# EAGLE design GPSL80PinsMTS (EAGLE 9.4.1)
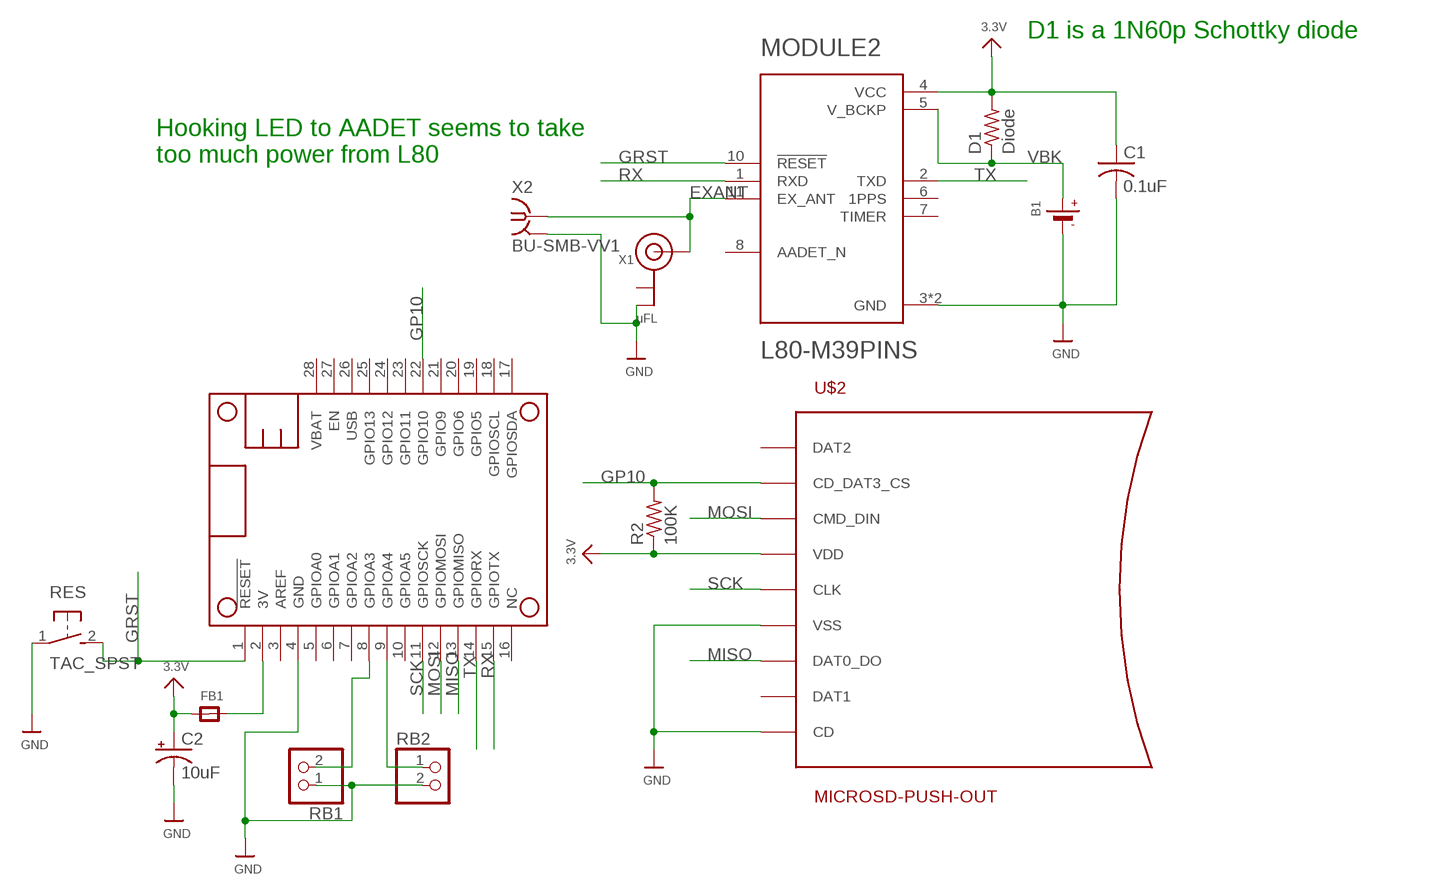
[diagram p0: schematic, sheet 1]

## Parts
B1  MICROBUILDER_BATTERYCR1220_2  [MICROBUILDER_CR1220-2]
C1  0.1uF  C-US025-025X050  [C025-025X050]
C2  10uF  CPOL-USE2.5-5V  [E2,5-4R]
D1  Diode  R-US_0204/2V  [0204V]
FB1  MICROBUILDER_FERRITE0805  [MICROBUILDER_0805]
MODULE2  L80-M39PINS  [L80PINS]
MS2  MICROBUILDER_FEATHERWINGLITE  [FEATHERWING_LITE]
R2  100K  R-US_0204/2V  [0204V]
RB1  PINHD-1X2  [1X02]
RB2  PINHD-1X2  [1X02]
RES  TAC_SPST  [TACTILE-SPST]
U$2  MICROSD-PUSH-OUT  [MICROSD-PUSH-OUT]
X1  uFL  ANTENNA_U.FL  [U.FL]
X2  BU-SMB-VV1  [BU-SMB-V1]

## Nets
3.3V: C1.1 C2.+ D1.2 FB1.1 MODULE2.4(VCC) R2.1 U$2.4(VDD)
3V: FB1.2 MS2.2(3V)
EXANT: MODULE2.11(EX_ANT) X1.3(SIGNAL) X2.1
GND: B1.- C1.2 C2.- MODULE2.3(GND) MODULE2.12(GND) MS2.4(GND) RB1.1 RB2.2 RES.1 U$2.6(VSS) U$2.CD U$2.G1(VSS) U$2.G2(VSS) U$2.G3(VSS) U$2.G4(VSS) X1.2(GND) X2.2 X2.3 X2.4 X2.5
GP10: MS2.22(GPIO10) R2.2 U$2.2(CD_DAT3_CS)
GRST: MODULE2.10(!RESET) MS2.1(!RESET) RES.2
MISO: MS2.13(GPIOMISO) U$2.7(DAT0_DO)
MOSI: MS2.12(GPIOMOSI) U$2.3(CMD_DIN)
N$1: MS2.8(GPIOA3) RB1.2
N$2: MS2.9(GPIOA4) RB2.1
RX: MODULE2.1(RXD) MS2.15(GPIOTX)
SCK: MS2.11(GPIOSCK) U$2.5(CLK)
TX: MODULE2.2(TXD) MS2.14(GPIORX)
VBK: B1.+ D1.1 MODULE2.5(V_BCKP)
Unconnected: MODULE2.6(1PPS) MODULE2.7(TIMER) MODULE2.8(AADET_N) MS2.3(AREF) MS2.5(GPIOA0) MS2.6(GPIOA1) MS2.7(GPIOA2) MS2.10(GPIOA5) MS2.16(NC) MS2.17(GPIOSDA) MS2.18(GPIOSCL) MS2.19(GPIO5) MS2.20(GPIO6) MS2.21(GPIO9) MS2.23(GPIO11) MS2.24(GPIO12) MS2.25(GPIO13) MS2.26(USB) MS2.27(EN) MS2.28(VBAT) U$2.1(DAT2) U$2.8(DAT1) X1.1(GND)

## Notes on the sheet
- D1 is a 1N60p Schottky diode
- Hooking LED to AADET seems to take 
  too much power from L80

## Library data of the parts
B1 = Adafruit Ultimate GPS FeatherWing:MICROBUILDER_BATTERY: CR1220 SMT - Digikey: 3001K-ND
C1 = rcl:C-US: CAPACITOR, American symbol; SPICEPREFIX: C
C2 = rcl:CPOL-US: POLARIZED CAPACITOR, American symbol; SPICEPREFIX: C
D1 R2 = rcl:R-US_: RESISTOR, American symbol; SPICEPREFIX: R
FB1 = Adafruit Ultimate GPS FeatherWing:MICROBUILDER_FERRITE: Ferrite Bead
MODULE2 = MTS_Custom:L80-M39: GPS Receiver 1575.42MHz 3.3V 12-Pin
MS2 = MTS_Custom:MICROBUILDER_FEATHERWING
RB1 RB2 = MTS_Custom:PINHD-1X2: PIN HEADER
RES = MTS_Custom:TAC_SPST: Tactile switch SPST 7mm lead spacing
U$2 = microsd:MICROSD-PUSH-OUT: T-Flash Push-Out Micro SD Card Reader 14.75mm x 14.5mm SMD with external pins
X1 = microbuilder:ANTENNA_U.FL: U.FL Antenna Connector
X2 = MTS_Custom:BU-SMB-V: FEMALE SMB CONNECTOR

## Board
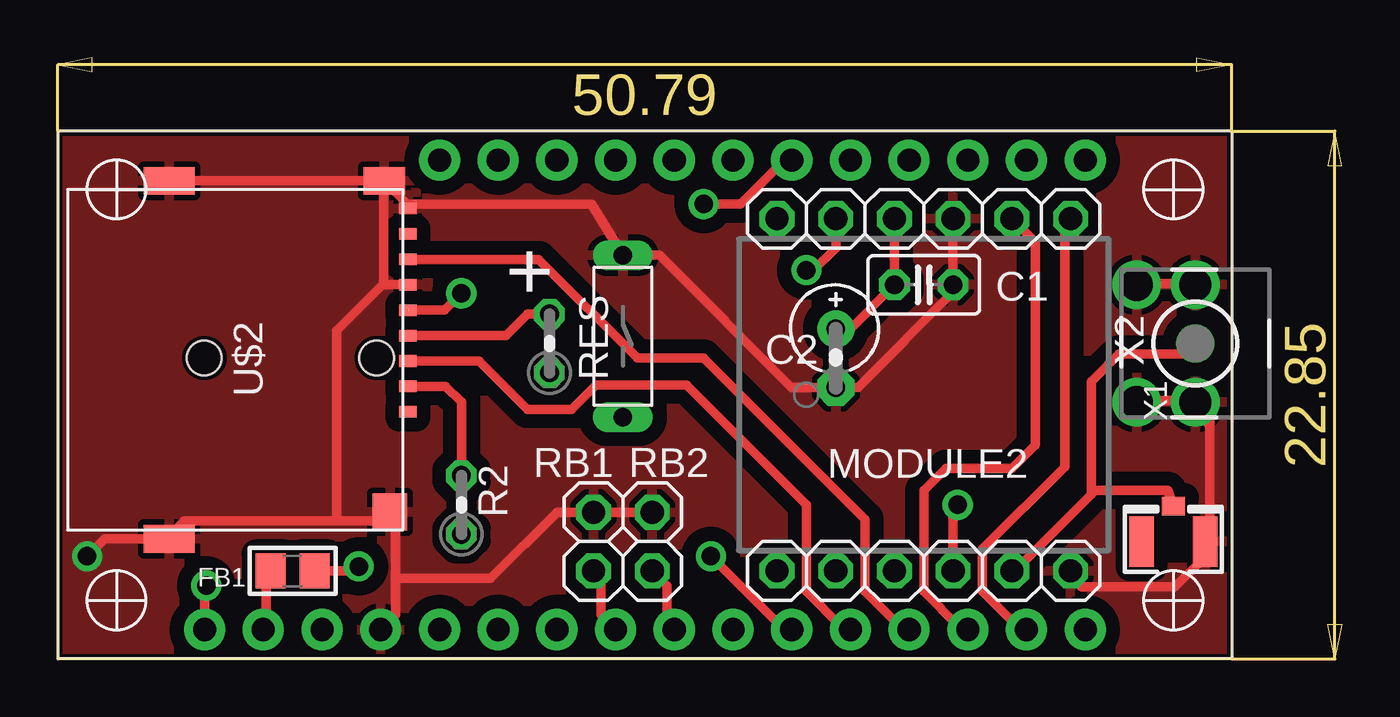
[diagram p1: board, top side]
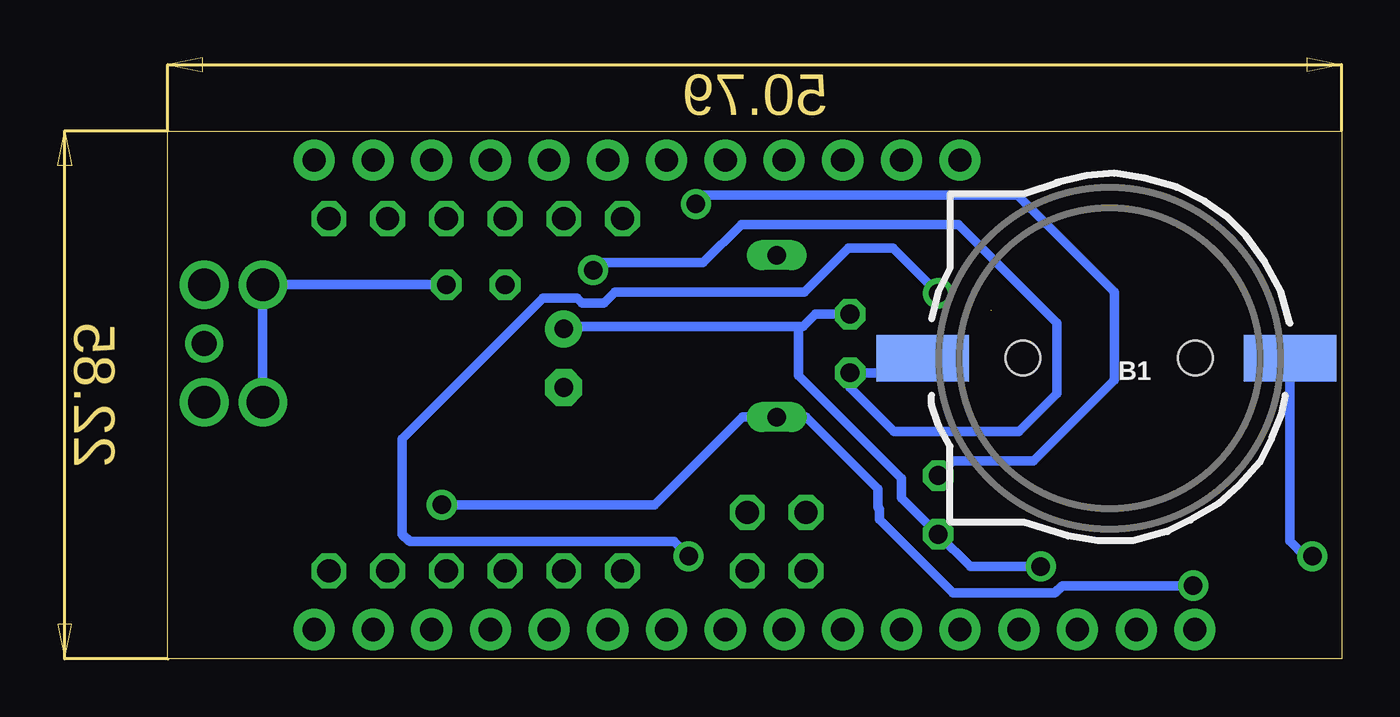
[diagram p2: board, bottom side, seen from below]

Size 55.54 x 26.02 mm. Coordinates in mm from the lower left corner, seen from the top.
Outline: 0,0 50.79,0 50.79,22.85 0,22.85 0,0
Copper layers (1*16): Top 0.035mm / dielectric 1.5mm / Bottom 0.035mm
Design rules "MTS": minimum track width 16mil, minimum drill 12mil, track to track 24mil, track to pad 16mil, pad to pad 6mil, via to via 6mil, smd to smd 0mil, copper to edge 8mil, drill to drill 10mil, minimum pad ring 10mil, minimum via ring 10mil, stop-mask expansion 2mil, vias tented up to drill 25mil, thermal gap 10mil

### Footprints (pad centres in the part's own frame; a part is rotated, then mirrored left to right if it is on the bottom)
MICROBUILDER_CR1220-2 = smd 4 x 2: + 8.29,0; - -7.6,0 | hole 1.5: 3.95,0; -3.5,0
C025-025X050 = drill 0.813 octagon: 1 -1.27,0; 2 1.27,0
E2,5-4R = drill 0.813 pad 1.6: + -1.27,0 | drill 0.813 pad 1.6 octagon: - 1.27,0
0204V = drill 0.813 octagon: 1 -1.27,0; 2 1.27,0
MICROBUILDER_0805 = smd 1.3 x 1.5: 1 -0.95,0; 2 0.95,0
L80PINS = drill 1 octagon: 1 7.62,-6.35; 2 7.62,-3.81; 3 7.62,-1.27; 4 7.62,1.27; 5 7.62,3.81; 6 7.62,6.35; 7 -7.62,6.35; 8 -7.62,3.81; 9 -7.62,1.27; 10 -7.62,-1.27; 11 -7.62,-3.81; 12 -7.62,-6.35
FEATHERWING_LITE = drill 1 pad 1.778: 1 6.35,1.27; 2 8.89,1.27; 3 11.43,1.27; 4 13.97,1.27; 5 16.51,1.27; 6 19.05,1.27; 7 21.59,1.27; 8 24.13,1.27; 9 26.67,1.27; 10 29.21,1.27; 11 31.75,1.27; 12 34.29,1.27; 13 36.83,1.27; 14 39.37,1.27; 15 41.91,1.27; 16 44.45,1.27; 17 44.45,21.59; 18 41.91,21.59; 19 39.37,21.59; 20 36.83,21.59; 21 34.29,21.59; 22 31.75,21.59; 23 29.21,21.59; 24 26.67,21.59; 25 24.13,21.59; 26 21.59,21.59; 27 19.05,21.59; 28 16.51,21.59
1X02 = drill 1 octagon: 1 -1.27,0; 2 1.27,0
TACTILE-SPST = drill 0.8 long: 1 0,3.5; 2 0,-3.5
MICROSD-PUSH-OUT = smd 0.5 x 0.75: 1 9.625,0.225; 2 8.525,0.225; 3 7.425,0.225; 4 6.325,0.225; 5 5.225,0.225; 6 4.125,0.225; 7 3.025,0.225; 8 1.925,0.225; CD 0.825,0.225 | smd 1.2 x 1.8: G1 -0.375,-0.8 | smd 1.2 x 2.2: G2 -0.375,-10.1; G4 15.125,-10.1 | smd 1.6 x 1.5: G3 13.95,-0.55
U.FL = smd 2.2 x 1.05: 1 0,1.375; 2 0,-1.375 | smd 0.8 x 1: 3 1.525,0
BU-SMB-V1 = drill 1.1: 1 0,0 | drill 1.4: 2 -2.54,2.54; 3 2.54,2.54; 4 2.54,0; 5 -2.54,0

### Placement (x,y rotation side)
B1  9.84,13.02 180 bottom
C1  37.47,16.19 0 top
C2  33.66,13.02 270 top
D1  21.27,13.65 90 top
FB1  10.16,3.81 180 top
MODULE2  37.47,11.43 90 top
MS2  0,0 0 top
R2  17.46,6.67 90 top
RB1  23.18,5.08 270 top
RB2  25.72,5.08 90 top
RES  24.45,13.97 0 top
U$2  14.92,20.32 270 top
X1  48.26,5.08 90 top
X2  49.21,13.65 90 top

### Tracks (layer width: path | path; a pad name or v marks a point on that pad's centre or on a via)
3.3V  (via drill 0.8)
  Top 0.406: MODULE2.4 C1.1 34.29,14.29 C2.+ | U$2.4 19.39,13.99 20.32,14.92 D1.2 | FB1.1 12.7,3.81 12.9,4.01 v13.02,4.01
  Bottom 0.406: v13.02,4.01 16.07,4.01 R2.1 19.04,6.97 19.04,7.82 23.5,12.28 23.5,14.38 | C2.+ 33.56,14.38 23.5,14.38 | 23.5,14.38 23.3,14.38 22.76,14.92 D1.2
3V
  Top 0.406: FB1.2 9.02,3.43 9.02,1.4 MS2.2
EXANT
  Top 0.406: 44.7,7.11 41.53,3.94 MODULE2.11 | 44.7,7.11 44.9,7.3 48.03,7.3 X1.3 | 44.7,7.11 44.7,12 45.91,13.21 48.77,13.21 X2.1
GND  (via drill 0.8)
  Top 0.406: 49.66,4.95 49.66,4.45 48.32,3.11 44.28,3.11 MODULE2.12 | 12.06,5.97 5.46,5.97 4.95,5.46 U$2.G4 2.02,5.2 v1.27,4.45 | 12.06,5.97 14.1,5.97 U$2.G3 14.61,6.14 14.61,3.49 | U$2.G1 14.1,20.19 14.1,16.26 12.06,14.22 12.06,5.97 | 15.11,19.68 14.61,20.19 U$2.G1 | U$2.G2 4.95,20.7 14.1,20.7 U$2.G1 | 15.11,19.68 23.09,19.68 RES.1 26.03,17.47 31.75,11.75 C2.- 34.61,11.75 38.73,15.88 C1.2 MODULE2.3 | 15.11,19.68 U$2.CD | X2.2 46.74,11.18 48.77,11.18 X2.5 | 49.78,10.16 49.28,10.67 X2.5 | X2.3 46.74,16.26 48.77,16.26 X2.4 | U$2.6 14.1,16.19 | MS2.4 14.61,1.91 14.61,3.49 | RB2.2 RB1.1 21.59,6.35 18.73,3.49 14.61,3.49 | X2.5 49.85,10.48 49.85,5.71
  Bottom 0.406: B1.- 2.24,5.1 1.59,4.45 v1.27,4.45 | C1.2 X2.3 X2.2
  pour Top: 0,22.86 0,0 50.8,0 50.8,22.86
GP10  (via drill 0.8)
  Top 0.406: MS2.22 31.43,21.59 29.53,19.68 v27.94,19.68 | U$2.2 16.78,11.79 17.46,11.11 R2.2
  Bottom 0.406: v27.94,19.68 27.56,20.07 14.03,20.07 9.84,15.88 9.84,12.06 13.34,8.57 16.83,8.57 R2.2
GRST  (via drill 0.8)
  Top 0.406: MS2.1 6.35,3.17 v6.42,3.17 | v38.93,6.67 38.73,6.47 MODULE2.10
  Bottom 0.406: v38.93,6.67 29.72,6.67 25.92,10.47 RES.2 23.18,10.48 20.05,7.35 20.05,6.55 20,6.5 20,6.03 16.83,2.86 12.41,2.86 12.09,3.17 v6.42,3.17
MISO
  Top 0.406: MS2.13 36.58,1.27 34.92,2.93 34.92,6.03 27.94,13.02 25.08,13.02 20.8,17.3 U$2.7
MOSI
  Top 0.406: MS2.12 33.91,1.4 32.38,2.92 32.38,6.67 27.2,11.85 23.28,11.85 22.23,10.79 20.32,10.79 18.22,12.89 U$2.3
N$1
  Top 0.406: MS2.8 23.5,1.91 23.5,3.49 RB1.2
N$2
  Top 0.406: MS2.9 26.35,1.59 26.35,3.17 RB2.1
RX
  Top 0.406: MODULE2.1 43.56,18.67 43.56,8.32 40.01,4.76 40.01,2.92 41.53,1.4 MS2.15
SCK  (via drill 0.8)  (1 unrouted)
  Top 0.406: MS2.11 31.43,1.27 v28.26,4.45 | v17.46,15.83 16.73,15.1 15.17,15.1 15.15,15.08
  Bottom 0.406: v17.46,15.83 19.41,17.78 21.34,17.78 23.25,15.88 31.43,15.88 31.91,15.4 32.86,15.4 33.08,15.61 34.55,15.61 40.64,9.53 40.64,5.4 40.32,5.08 28.89,5.08 v28.26,4.45
TX
  Top 0.406: MODULE2.2 42.29,18.03 42.29,9.27 41.27,8.26 38.42,8.26 37.47,7.3 37.47,2.92 38.99,1.4 MS2.14
VBK  (via drill 0.8)
  Top 0.406: MODULE2.5 33.66,17.78 32.7,16.83 v32.38,16.83
  Bottom 0.406: v32.38,16.83 32.07,17.14 27.62,17.14 25.97,18.8 16.57,18.8 12.32,14.54 12.32,11.49 13.97,9.84 19.37,9.84 21.27,11.75 D1.1 18.77,12.38 B1.+

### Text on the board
tPlace: +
